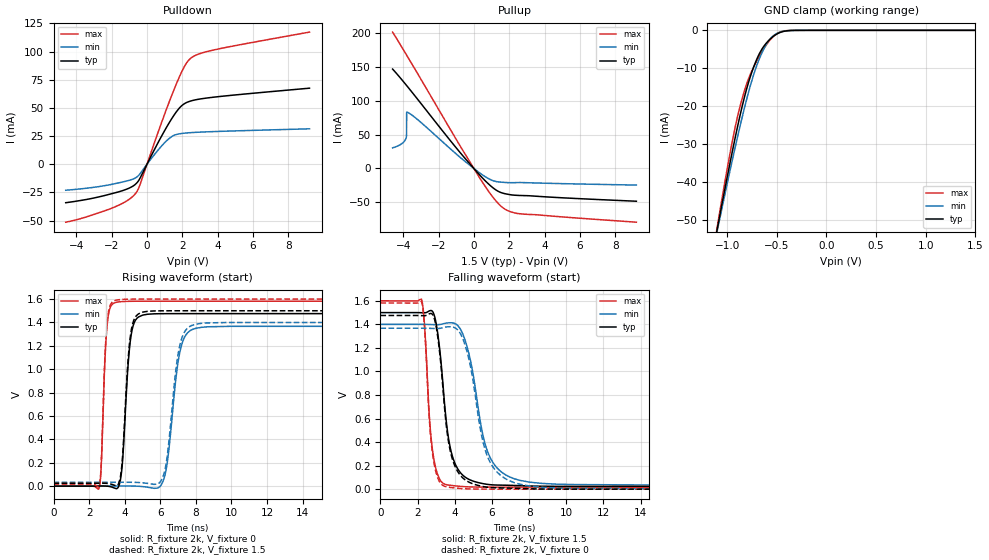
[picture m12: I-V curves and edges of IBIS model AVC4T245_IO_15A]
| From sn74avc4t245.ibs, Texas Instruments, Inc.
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[Model]   AVC4T245_IO_15A
Model_type  I/O
Vinl=0.49
Vinh=1.04
Enable   Active-Low
Vref =   0
Rref =   2000
Cref =   15p
Vmeas =   0.75
| variable   typ   min   max
C_comp   5.20pF   4.57pF   5.81pF
| C_pullup   5.13pF   3.67pF   7.57pF
| C_pulldown   4.81pF   4.29pF   5.47pF
| C_tri-state   5.20pF   4.57pF   5.81pF
[Temperature Range]   40   100   -40
| Ambient temperature   25   85   -40
[Voltage range]   1.5   1.4   1.6
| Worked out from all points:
|   slope of the pulldown table from 0 to 0.225 V, typ, clamps not added: 32.1 ohm
|   slope of the pullup table from 0 to 0.225 V, typ, clamps not added: 33.9 ohm
|   GND clamp passes 1 mA (typ) near -0.50 V on its own axis
|   rising waveform, R_fixture 2k, V_fixture 0: 20-80 % time 356ps typ, 582ps min, 237ps max; typ from 0 V to 1.48 V
|   falling waveform, R_fixture 2k, V_fixture 1.5: 20-80 % time 628ps typ, 1ns min, 383ps max; typ from 1.5 V to 0.023 V
|   rising waveform, R_fixture 2k, V_fixture 1.5: 20-80 % time 352ps typ, 570ps min, 236ps max; typ from 0.023 V to 1.5 V
|   falling waveform, R_fixture 2k, V_fixture 0: 20-80 % time 629ps typ, 999ps min, 377ps max; typ from 1.48 V to 0 V
[GND Clamp]
| AVC4T245_IO_15A
|   Voltage   I(typ)   I(min)   I(max)
-4.6V     -600.6mA   -549.4mA   -665.2mA
-1.1V     -52.36mA   -52.84mA   -51.77mA
-1.075V   -48.9mA    -49.7mA    -47.87mA
-930mV    -29.64mA   -32.08mA   -26.89mA
-830mV    -18.03mA   -20.88mA   -16.26mA
-765mV    -12.07mA   -14.45mA   -11.48mA
-685mV    -6.658mA   -8.11mA    -7.261mA
-605mV    -3.351mA   -3.683mA   -3.806mA
-535mV    -1.602mA   -1.427mA   -1.608mA
-460mV    -500.6uA   -413.6uA   -383.6uA
-350mV    -38.76uA   -40.6uA    -15.38uA
1.5V      810.6pA    34.45nA    85.67pA
[Pulldown]
| AVC4T245_IO_15A
|   Voltage   I(typ)   I(min)   I(max)
-4.6V     -34.07mA   -23.01mA   -51.35mA
-1.875V   -25.58mA   -17.41mA   -38.17mA
-1.085V   -21.64mA   -14.57mA   -31.92mA
-625mV    -17.31mA   -11.83mA   -25.44mA
-415mV    -12.94mA   -8.777mA   -18.95mA
595mV     18.22mA    11.97mA    26.91mA
1.265V    37.01mA    23.01mA    55.56mA
1.7V      47.29mA    26.56mA    72.61mA
2.03V     52.78mA    27.45mA    84.03mA
2.5V      56.24mA    28.09mA    94.31mA
3.84V     59.63mA    29.04mA    101.6mA
9.2V      67.51mA    31.46mA    117.2mA
[Pullup]
| AVC4T245_IO_15A
|   Voltage   I(typ)   I(min)   I(max)
-4.6V     146.8mA    30.47mA    201.5mA
-4.1V     131.8mA    36.24mA    180.2mA
-3.85V    123.9mA    43.97mA    169.4mA
-3.81V    122.6mA    49.37mA    167.6mA
-3.805V   122.5mA    83.3mA     167.4mA
-3.785V   121.8mA    83.17mA    166.5mA
-3.155V   101.3mA    71.56mA    138.8mA
175mV     -5.197mA   -3.574mA   -7.497mA
980mV     -26.35mA   -16.94mA   -39.04mA
1.625V    -36.35mA   -20.39mA   -57.65mA
2.595V    -39.89mA   -20.78mA   -66.9mA
9.2V      -48.41mA   -24.54mA   -79.36mA
[Ramp]
| AVC4T245_IO_15A
| variable   typ   min   max
dV/dt_r   0.90/3.69E-10   0.83/5.93E-10   0.96/2.51E-10
dV/dt_f   0.90/6.39E-10   0.83/1.01E-09   0.96/3.92E-10
R_load = 2k
[Rising Waveform]
| AVC4T245_IO_15A
R_fixture =   2k
C_fixture =   0
L_fixture =   0
V_fixture =   0
V_fixture_min = 0
V_fixture_max = 0
|   Time   V(typ)   V(min)   V(max)
0s        19.4nV     97.73nV    508.8pV
2.565ns   914.7uV    -147.9uV   -15.62mV
3.005ns   -169.8uV   139.7uV    1.366V
3.505ns   -20.74mV   676.6uV    1.571V
4.365ns   1.294V     539.1uV    1.581V
5.015ns   1.463V     -3.901mV   1.582V
6.19ns    1.475V     56.69mV    1.582V
7.1ns     1.475V     1.147V     1.582V
7.98ns    1.475V     1.349V     1.582V
40ns      1.476V     1.367V     1.582V
[Falling Waveform]
| AVC4T245_IO_15A
R_fixture =   2k
C_fixture =   0
L_fixture =   0
V_fixture =   1.5
V_fixture_min = 1.4
V_fixture_max = 1.6
|   Time   V(typ)   V(min)   V(max)
0s        1.5V       1.4V       1.6V
2.21ns    1.499V     1.4V       1.615V
2.805ns   1.51V      1.398V     329.1mV
3.13ns    1.27V      1.398V     104.1mV
3.55ns    569mV      1.411V     38.42mV
3.92ns    257.3mV    1.411V     29.79mV
4.57ns    101.3mV    1.26V      20.86mV
5.885ns   38.53mV    274.7mV    17.36mV
7.505ns   29.8mV     74.76mV    17.21mV
40ns      23.49mV    32.45mV    17.19mV
[Rising Waveform]
| AVC4T245_IO_15A
R_fixture =   2k
C_fixture =   0
L_fixture =   0
V_fixture =   1.5
V_fixture_min = 1.4
V_fixture_max = 1.6
|   Time   V(typ)   V(min)   V(max)
0s        23.49mV    32.45mV    17.19mV
2.56ns    24.38mV    32.33mV    -42.69uV
3ns       23.3mV     32.62mV    1.382V
3.5ns     3.561mV    33.11mV    1.59V
4.34ns    1.306V     32.84mV    1.599V
5.005ns   1.488V     28.55mV    1.6V
6.175ns   1.5V       91.22mV    1.6V
7.065ns   1.5V       1.182V     1.6V
7.925ns   1.5V       1.382V     1.6V
40ns      1.5V       1.4V       1.6V
[Falling Waveform]
| AVC4T245_IO_15A
R_fixture =   2k
C_fixture =   0
L_fixture =   0
V_fixture =   0
V_fixture_min = 0
V_fixture_max = 0
|   Time   V(typ)   V(min)   V(max)
0s        1.476V     1.367V     1.582V
2.21ns    1.474V     1.367V     1.596V
2.8ns     1.485V     1.365V     308.7mV
3.125ns   1.247V     1.365V     80.73mV
3.53ns    564.1mV    1.377V     21.02mV
3.905ns   239.5mV    1.377V     11.94mV
4.55ns    80.35mV    1.227V     3.348mV
5.84ns    14.95mV    249.3mV    163.7uV
7.505ns   5.782mV    41.92mV    16.31uV
40ns      65.58nV    546.5nV    57.64nV
